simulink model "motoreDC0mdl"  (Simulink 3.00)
settings: Solver=ode45  StartTime=0.0  StopTime=10.0  RelTol=1e-6  AbsTol=1e-6
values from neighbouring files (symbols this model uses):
  bme = Ic0*KI/Wmax    (= 1.40697764938e-05)    [motoreDC0.m]
  Ime0 = 0    [motoreDC0.m]
  Jme = 7.06*mg*m^2    (= 7.06e-06)    [motoreDC0.m]
  KI = Cmax/Imax    (= 0.0452697095436)    [motoreDC0.m]
  Lme = 2.63*mHenry    (= 0.00263)    [motoreDC0.m]
  Rme0 = Vn/Imax    (= 2.48962655602)    [motoreDC0.m]
  Tcsim = 1*msec    (= 0.001)    [motoreDC0.m]
  th0 = 0    [motoreDC0.m]
  Wme0 = 0    [motoreDC0.m]
libraries: simulink3 x2

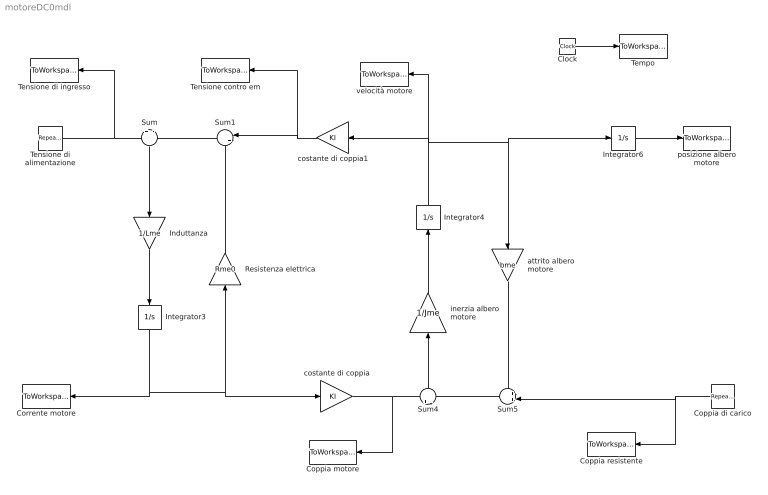
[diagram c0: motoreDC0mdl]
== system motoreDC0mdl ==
  Clock : Clock
  Coppia motore : ToWorkspace  VariableName=Cm  SampleTime=Tcsim  SaveFormat=Matrix
  Coppia resistente : ToWorkspace  VariableName=Cr  SampleTime=Tcsim  SaveFormat=Matrix
  Coppia di carico : simulink3/Sources/Repeating Sequence  Orientation=left  rep_seq_t=TABTEMPI  rep_seq_y=TABCR
  Corrente motore : ToWorkspace  VariableName=Ime  SampleTime=Tcsim  SaveFormat=Matrix
  Induttanza : Gain  Orientation=down  Gain=1/Lme  SaturateOnIntegerOverflow=on
  Integrator3 : Integrator  Orientation=down  ExternalReset=none  InitialConditionSource=internal  InitialCondition=Ime0  LimitOutput=off  UpperSaturationLimit=inf  LowerSaturationLimit=-inf  ShowSaturationPort=off  ShowStatePort=off  AbsoluteTolerance=auto
  Integrator4 : Integrator  Orientation=up  ExternalReset=none  InitialConditionSource=internal  InitialCondition=Wme0  LimitOutput=off  UpperSaturationLimit=inf  LowerSaturationLimit=-inf  ShowSaturationPort=off  ShowStatePort=off  AbsoluteTolerance=auto
  Integrator6 : Integrator  ExternalReset=none  InitialConditionSource=internal  InitialCondition=th0  LimitOutput=off  UpperSaturationLimit=inf  LowerSaturationLimit=-inf  ShowSaturationPort=off  ShowStatePort=off  AbsoluteTolerance=auto
  Resistenza elettrica : Gain  Orientation=up  Gain=Rme0  SaturateOnIntegerOverflow=on
  Sum : Sum  Orientation=down  Inputs=+|-  SaturateOnIntegerOverflow=on
  Sum1 : Sum  Orientation=left  Inputs=|++  SaturateOnIntegerOverflow=on
  Sum4 : Sum  Orientation=up  Inputs=+|-  SaturateOnIntegerOverflow=on
  Sum5 : Sum  Orientation=left  Inputs=++|  SaturateOnIntegerOverflow=on
  Tempo : ToWorkspace  VariableName=t  SampleTime=Tcsim  SaveFormat=Matrix
  Tensione contro em : ToWorkspace  VariableName=Vcem  SampleTime=Tcsim  SaveFormat=Matrix
  Tensione di ingresso : ToWorkspace  VariableName=Vi  SampleTime=Tcsim  SaveFormat=Matrix
  Tensione di alimentazione : simulink3/Sources/Repeating Sequence  rep_seq_t=TABTEMPI  rep_seq_y=TABVIN
  attrito albero motore : Gain  Orientation=down  Gain=bme  SaturateOnIntegerOverflow=on
  costante di coppia : Gain  Gain=KI  SaturateOnIntegerOverflow=on
  costante di coppia1 : Gain  Orientation=left  Gain=KI  SaturateOnIntegerOverflow=on
  inerzia albero motore : Gain  Orientation=up  Gain=1/Jme  SaturateOnIntegerOverflow=on
  posizione albero motore : ToWorkspace  VariableName=th  SampleTime=Tcsim  SaveFormat=Matrix
  velocità motore : ToWorkspace  VariableName=Wme  SampleTime=Tcsim  SaveFormat=Matrix
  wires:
  Tensione di alimentazione/1 -> Sum/1, Tensione di ingresso/1
  Sum/1 -> Induttanza/1
  Induttanza/1 -> Integrator3/1
  Sum1/1 -> Sum/2
  Integrator3/1 -> Corrente motore/1, costante di coppia/1, Resistenza elettrica/1
  Resistenza elettrica/1 -> Sum1/2
  Sum4/1 -> inerzia albero motore/1
  inerzia albero motore/1 -> Integrator4/1
  Sum5/1 -> Sum4/2
  attrito albero motore/1 -> Sum5/1
  Coppia di carico/1 -> Coppia resistente/1, Sum5/2
  Integrator4/1 -> velocità motore/1, attrito albero motore/1, Integrator6/1, costante di coppia1/1
  Integrator6/1 -> posizione albero motore/1
  costante di coppia/1 -> Sum4/1, Coppia motore/1
  costante di coppia1/1 -> Sum1/1, Tensione contro em/1
  Clock/1 -> Tempo/1
